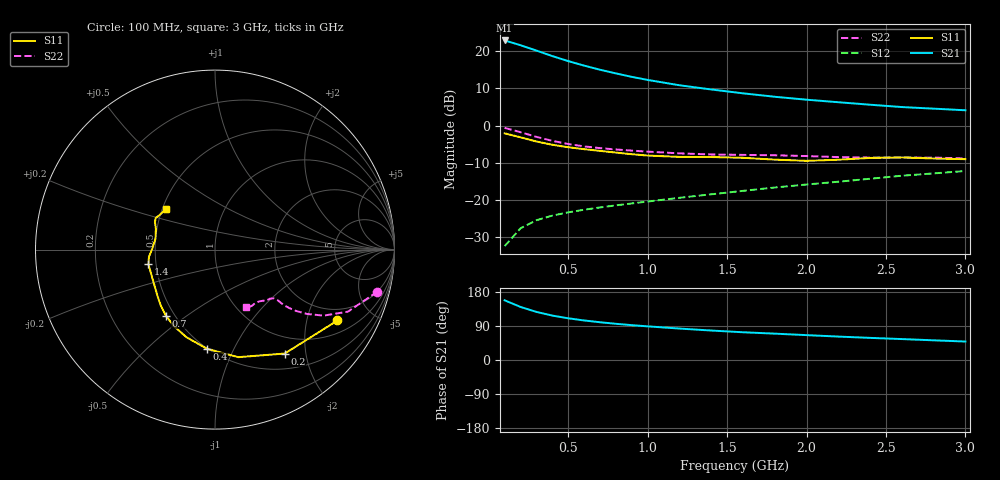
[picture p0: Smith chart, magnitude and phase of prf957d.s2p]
! Filename:  PRF957D.S2P  Version:  3.0
! Philips part #:  PRF957  Date:  Nov 1998
! Bias condition:  Vce=3V, Ic=5mA
#  MHz  S  MA  R 50
! Freq  S11  S21  S12  S22
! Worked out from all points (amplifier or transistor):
!   20 points, 100 MHz to 3 GHz, reference 50 ohm
!   highest |S21| = 22.9 dB at 100 MHz (marker M1)
!   |S21| within 3 dB of that: start of sweep to 319.3 MHz
!   unconditionally stable (mu >= 1): 1.403 GHz to end of sweep
!   at 400 MHz: K = 0.48, MSG = 21.4 dB, |S12| = -24.1 dB
!   at 1.2 GHz: K = 0.97, MSG = 15.1 dB, |S12| = -19.4 dB
!   at 3 GHz: K = 1.06, MAG = 6.7 dB, |S12| = -12.2 dB
!   S11 on the Smith chart (normalised r, x): 100 MHz: 1.47, -3.08; 200 MHz: 0.72, -1.63; 400 MHz: 0.50, -0.79; 700 MHz: 0.45, -0.42; 1.4 GHz: 0.45, -0.09; 3 GHz: 0.52, +0.27
100  0.7885 -30.1  13.9 157.5  0.02416 74.6  0.9344 -14.6
200  0.6975 -56.1  12.01 140.1  0.04197 64.1  0.8175 -25.0
300  0.6131 -77.8  10.17 126.9  0.05384 58.1  0.7079 -31.3
400  0.5542 -94.7  8.582 117.3  0.06206 55.1  0.6254 -35.0
500  0.5136 -108.0  7.352 110.1  0.06868 54.4  0.5673 -37.1
600  0.4837 -118.3  6.396 104.3  0.07445 54.5  0.5273 -38.2
700  0.4587 -126.6  5.632 99.6  0.07994 55.3  0.4997 -38.8
800  0.4354 -133.7  5.027 95.6  0.0852 56.4  0.4793 -38.9
900  0.414 -140.3  4.516 92.0  0.09042 57.7  0.4626 -38.9
1000  0.3971 -146.8  4.107 88.8  0.09592 59.1  0.4484 -39.0
1200  0.381 -158.6  3.487 83.0  0.1076 61.5  0.4249 -39.8
1400  0.3796 -167.5  3.06 77.8  0.1199 63.5  0.4106 -41.8
1600  0.3705 -173.7  2.715 73.2  0.1334 65.5  0.4053 -43.8
1800  0.3502 179.5  2.442 69.6  0.1481 67.0  0.4007 -45.2
2000  0.3372 169.9  2.23 65.6  0.1623 68.3  0.3909 -46.8
2200  0.3491 160.6  2.063 61.8  0.1771 69.2  0.3788 -49.6
2400  0.3689 155.2  1.91 58.4  0.1938 69.7  0.373 -53.5
2600  0.3745 151.9  1.777 55.2  0.213 70.0  0.3744 -56.9
2800  0.3626 147.4  1.691 51.9  0.2288 70.5  0.3726 -59.3
3000  0.355 139.8  1.608 48.7  0.2465 70.9  0.3636 -62.0
